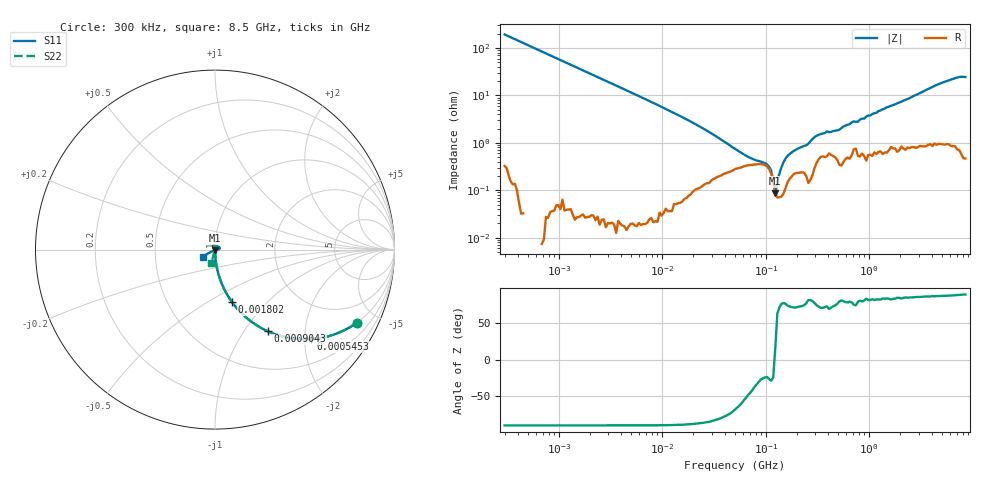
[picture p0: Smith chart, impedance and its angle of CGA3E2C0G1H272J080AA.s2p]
! S-parameter Generated by TDK Corporation
! Copyright(C) 2015 TDK Corporation.
! All Rights Reserved.
! TDK P/N: CGA3E2C0G1H272J080AA (Multilayer Ceramic Chip Capacitors)
! Property: C=2.7nF
! Size(LxWxT): 1.6x0.8x0.8mm, 0.063x0.031x0.031inches
! Model Type: s2p (Touchstone File Format Version 1.0)
! Frequency: DC=Yes Start=0.3MHz Stop=8500MHz 225points Log-sweep
! Note:
! Model Generated on Jun. 23, 2015
! Hash(MD5):
! Port Assignments:
!  1 ---| |--- 2
! Applicable Conditions:
!  Temperature = 25 degC
!  DC Bias Voltage = 0 V
!  Small Signal Operation
! Terms and conditions regarding TDK Simulation Models
! (1)This simulation model is being provided solely for informational purposes. Please refer to the specifications of the products in terms of detailed characteristics of such products.
! (2)In no event shall TDK Corporation of any of its subsidiaries be liable for any loss or damage arising, directly or indirectly,
!  From any information contained in this simulation model, including, but not limited to loss or damages arising from any inaccuracies, omissions or errors in connection with such information.
! (3)Any and all copyrights on this simulation model are owned by TDK Corporation.
!  Duplication or redistribution of this simulation model without prior written permission from TDK Corporation is prohibited.
! (4)This simulation model is subject to any modification or change without any prior notice.
! (5)Neither TDK Corporation nor any of its subsidiaries shall make any warranty, express or implied,
!  Including but not limited to the correctness, implied warranties of merchantability and fitness for a particular purpose with respect to this simulation models.
! (6)The use of this simulation model shall be deemed to have consented to the terms and conditions hereof.
# MHz S MA R 50
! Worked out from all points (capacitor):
!   224 points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, 300 kHz to 8.5 GHz, reference 50 ohm
!   read as one part in series: C = 2.74 nF near 314.1 kHz
!   lowest |Z| = 85.8 mohm at 123.8 MHz (marker M1)
!   series resonance near 122.4 MHz, so ESL is about 620 pH
!   S11 on the Smith chart (normalised r, x): 300 kHz: 1.00, -3.87; 545.3 kHz: 1.00, -2.14; 904.3 kHz: 1.00, -1.29; 1.802 MHz: 1.00, -0.65; 8.5 GHz: 0.88, -0.07
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0.3  0.8885 -27.3  0.4589 62.6  0.4589 62.7  0.8885 -27.4
0.5453461  0.7302 -43.0  0.6823 47.0  0.6826 47.0  0.7301 -43.2
0.9042579  0.541 -57.2  0.8407 32.8  0.8408 32.8  0.5408 -57.2
1.72111  0.3202 -71.3  0.9471 18.7  0.9472 18.7  0.32 -71.3
1.802081  0.3073 -72.1  0.9514 17.9  0.9515 17.9  0.3071 -72.1
9.430415  0.06056 -86.4  0.9977 3.4  0.9979 3.4  0.06039 -86.2
51.67171  0.007646 -87.6  0.9965 0.2  0.9966 0.3  0.01114 -67.0
123.7646  0.003614 -105.5  0.9969 -0.3  0.9968 -0.3  0.006449 -108.7
283.1228  0.002177 -152.7  0.9938 -1.3  0.9935 -1.3  0.00368 130.9
310.3886  0.0004378 -115.3  0.9925 -1.5  0.9923 -1.5  0.003992 86.4
408.9767  0.003169 -9.7  0.9912 -1.8  0.99 -1.8  0.002444 35.3
469.456  0.0001653 130.7  0.9915 -2.1  0.991 -2.0  0.00283 -38.3
743.4462  0.003363 -12.1  0.9894 -3.1  0.9893 -3.0  0.005579 7.1
1025.67  0.002126 -0.9  0.9894 -4.3  0.9901 -4.3  0.0008933 -111.1
1073.923  0.002621 6.9  0.9899 -4.4  0.9906 -4.5  0.005083 97.0
1290.729  0.00496 25.8  0.9894 -5.4  0.9884 -5.4  0.0008502 98.4
1551.304  0.003631 6.2  0.9882 -6.5  0.9876 -6.4  0.004205 77.4
1952.199  0.003033 28.6  0.9878 -8.0  0.9875 -8.1  0.0008441 33.6
2044.041  0.003756 13.1  0.9875 -8.3  0.987 -8.4  0.004362 1.2
5367.404  0.02822 23.6  0.9831 -21.7  0.982 -21.6  0.02479 105.1
7404.957  0.005677 -119.3  0.9835 -29.8  0.9829 -29.6  0.007605 -118.2
8500  0.07583 -149.2  0.9811 -34.1  0.981 -34.1  0.08021 -106.7
